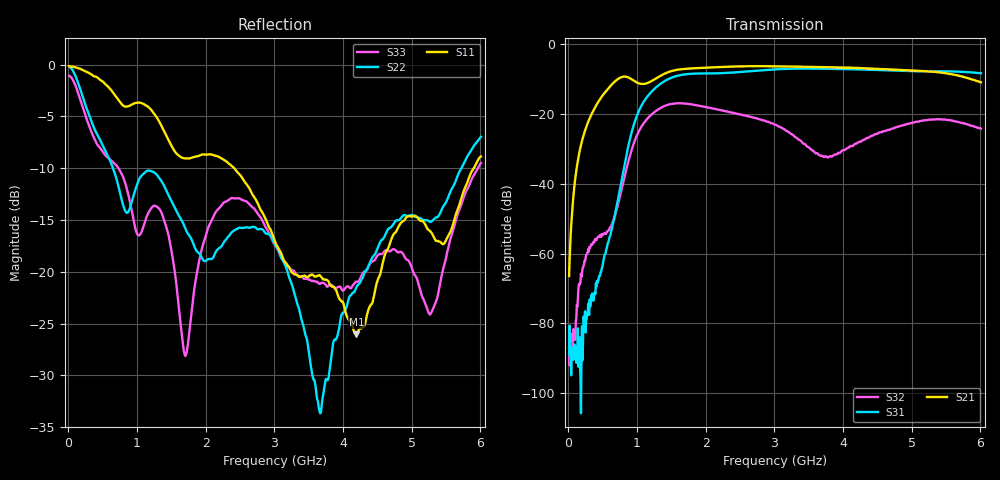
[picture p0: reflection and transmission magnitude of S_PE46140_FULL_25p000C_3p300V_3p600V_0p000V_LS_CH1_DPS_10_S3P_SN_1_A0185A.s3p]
! Device ID: PE46140_FULL
! File Path: z:\PE46140\MajorStates\25p000C\3p300\LS_CH1_DPS_10\PE46140_FULL_25p000C_3p300V_3p600V_0p000V_LS_CH1_DPS_10_S3P_SN_1_A0185A.s3p
! Serial: 1
! Lot: A0185A
! Temp: 25.000C
! VDD: 3.300
! VSS: 0.000
! Control_Hi: 3.600
! Control_Lo: 0.000
! Logic State: LS_CH1_DPS_10
! Port 1: RFIN
! Port 2: RFOUT1
! Port 3: RFOUT2
! ThroughPath:1-2
! IDD: 0.0003111038
! ISS: -1.694e-007
! Comment:
#  Hz  S  RI  R  50
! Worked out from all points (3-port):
!   801 points, 10 MHz to 6.01 GHz, reference 50 ohm
!   strongest paths, dB at 10 MHz, 1.51 GHz, 3.01 GHz, 4.51 GHz, 6.01 GHz:
!     S21: -66.4, -7.6, -6.3, -7.1, -10.9
!     S31: -88.9, -9.5, -7.2, -7.4, -8.3
!     S32: -85.7, -17.1, -23.0, -25.5, -24.2
!   lowest |S11| = -26.0 dB at 4.195 GHz (marker M1), VSWR 1.10, Z = 45.6 + j1.96 ohm
!   |S11| at or under -10 dB: 2.416 GHz to 5.908 GHz (3.492 GHz wide, 83.9 % of centre)
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1e7  0.9808 -0.0667  0.000162 0.000446  4.42e-05 3.18e-05
     0.00014 0.000458  0.9749 -0.0928  -3.74e-06 -2.35e-05
     1.57e-05 -3.21e-05  -8.7e-06 5.09e-05  0.8808 -0.083
1.9e8  0.3768 -0.8689  -0.0164 0.0347  -3.33e-05 9.78e-05
       -0.0163 0.0347  -0.00354 -0.7301  -0.000423 0.000211
       -5.31e-07 2.88e-05  -0.000392 0.000255  -0.00323 -0.6511
6.55e8  -0.6996 -0.2037  0.2579 0.1077  0.00288 -0.000272
        0.2579 0.1083  -0.1492 0.2747  0.00128 0.00264
        0.00283 -0.000205  0.00129 0.00276  -0.1252 0.3123
1.2475e9  -0.4772 0.3292  0.1392 -0.2776  -0.2206 0.0534
          0.1397 -0.278  0.2349 0.1899  -0.055 0.0905
          -0.2208 0.0533  -0.055 0.0904  0.2022 0.0497
1.6975e9  -0.2448 0.254  -0.2536 -0.3656  0.2645 0.2592
          -0.2538 -0.3657  0.1627 -0.018  0.1055 -0.0944
          0.2647 0.2596  0.1057 -0.0943  -0.0386 -0.00857
1.9525e9  -0.2081 0.3042  -0.4256 -0.1727  0.3801 -0.0333
          -0.4257 -0.1729  0.1154 0.00275  -0.0552 -0.1165
          0.3805 -0.0334  -0.0553 -0.1166  0.0344 0.1275
3.01e9  0.0585 0.1274  0.1229 0.4679  -0.3762 -0.2235
        0.1222 0.4684  0.1004 -0.0915  0.0679 0.0185
        -0.3767 -0.2239  0.068 0.0184  0.1245 -0.0497
3.6625e9  -0.0241 0.093  0.4711 -0.000374  -0.3021 0.3295
          0.4713 8.89e-05  0.0187 -0.00961  -0.0238 -0.00947
          -0.302 0.3294  -0.0238 -0.00934  0.0852 -0.0201
4.195e9  -0.0451 0.0214  0.2149 -0.4057  0.1259 0.4189
         0.2156 -0.4057  0.0688 0.0487  0.0344 0.0152
         0.1261 0.419  0.0347 0.015  0.0875 -0.0193
6.01e9  -0.2267 -0.2797  0.1186 0.2589  -0.1837 -0.3362
        0.1182 0.2595  0.4454 0.0499  0.0615 0.00944
        -0.1853 -0.3372  0.0612 0.00921  0.3114 0.1239
